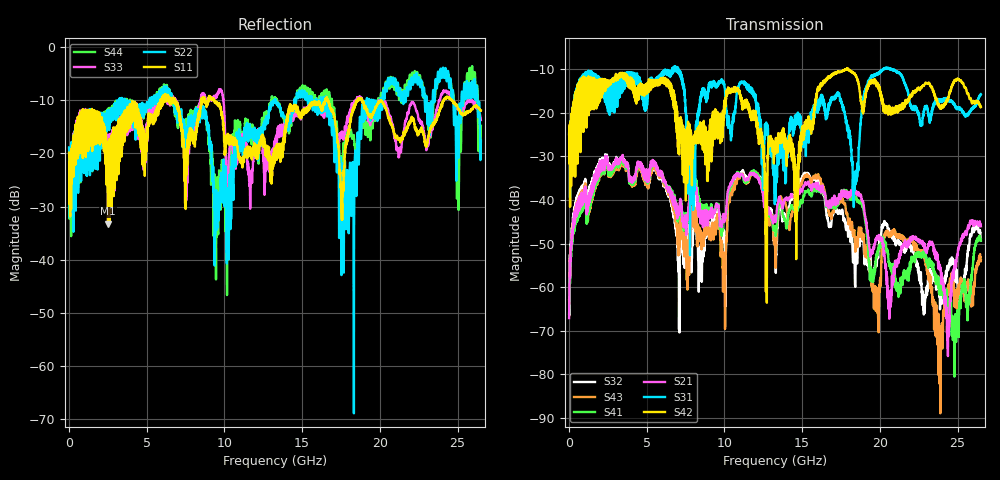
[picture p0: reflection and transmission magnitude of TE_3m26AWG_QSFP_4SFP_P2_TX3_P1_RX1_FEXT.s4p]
!Agilent Technologies,N5222A,MY51421691,A.10.00.00
!Agilent N5222A: A.10.00.00
!Date: Friday, January 30, 2015 12:36:29
!Correction: S11(Full 4 Port(1,2,3,4))
!S12(Full 4 Port(1,2,3,4))
!S13(Full 4 Port(1,2,3,4))
!S14(Full 4 Port(1,2,3,4))
!S21(Full 4 Port(1,2,3,4))
!S22(Full 4 Port(1,2,3,4))
!S23(Full 4 Port(1,2,3,4))
!S24(Full 4 Port(1,2,3,4))
!S31(Full 4 Port(1,2,3,4))
!S32(Full 4 Port(1,2,3,4))
!S33(Full 4 Port(1,2,3,4))
!S34(Full 4 Port(1,2,3,4))
!S41(Full 4 Port(1,2,3,4))
!S42(Full 4 Port(1,2,3,4))
!S43(Full 4 Port(1,2,3,4))
!S44(Full 4 Port(1,2,3,4))
!S4P File: Measurements: <S11,S12,S13,S14>,
!<S21,S22,S23,S24>,
!<S31,S32,S33,S34>,
!<S41,S42,S43,S44>:
# Hz S  dB  R 50.0
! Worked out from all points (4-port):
!   2650 points, 10 MHz to 26.5 GHz, reference 50 ohm
!   strongest paths, dB at 10 MHz, 6.63 GHz, 13.26 GHz, 19.88 GHz, 26.5 GHz:
!     S42: -24.9, -16.1, -29.5, -13.4, -18.6
!     S31: -24.9, -10.4, -34.1, -10.8, -15.7
!     S21: -67.1, -38.9, -44.1, -48.9, -46.0
!     S41: -66.2, -38.9, -46.4, -51.4, -49.0
!     S43: -63.0, -40.1, -50.7, -65.4, -53.8
!     S32: -60.6, -41.2, -49.5, -52.7, -49.3
!   lowest |S11| = -33.2 dB at 2.51 GHz (marker M1), VSWR 1.04, Z = 51 - j1.95 ohm
!   |S11| at or under -10 dB: start of sweep to 5.869 GHz; 9.355 GHz to 16.5 GHz (7.143 GHz wide, 55.3 % of centre); 20.09 GHz to 24.09 GHz (4.006 GHz wide, 18.1 % of centre)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
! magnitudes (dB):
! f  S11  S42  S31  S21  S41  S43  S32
! 10 MHz  -19.9  -24.9  -24.9  -67.1  -66.2  -63.0  -60.6
! 2.51 GHz  -33.2  -13.5  -19.7  -32.1  -33.0  -33.1  -31.9
! 9.97 GHz  -16.4  -18.7  -13.6  -44.6  -44.3  -52.1  -46.9
! 10.84 GHz  -18.6  -14.3  -14.8  -34.0  -33.7  -34.9  -34.8
! 12.68 GHz  -18.6  -45.1  -22.4  -42.5  -42.2  -43.2  -42.2
! 24.38 GHz  -9.6  -16.8  -17.1  -75.8  -64.2  -60.8  -55.8
! 26.5 GHz  -11.9  -18.6  -15.7  -46.0  -49.0  -53.8  -49.3
